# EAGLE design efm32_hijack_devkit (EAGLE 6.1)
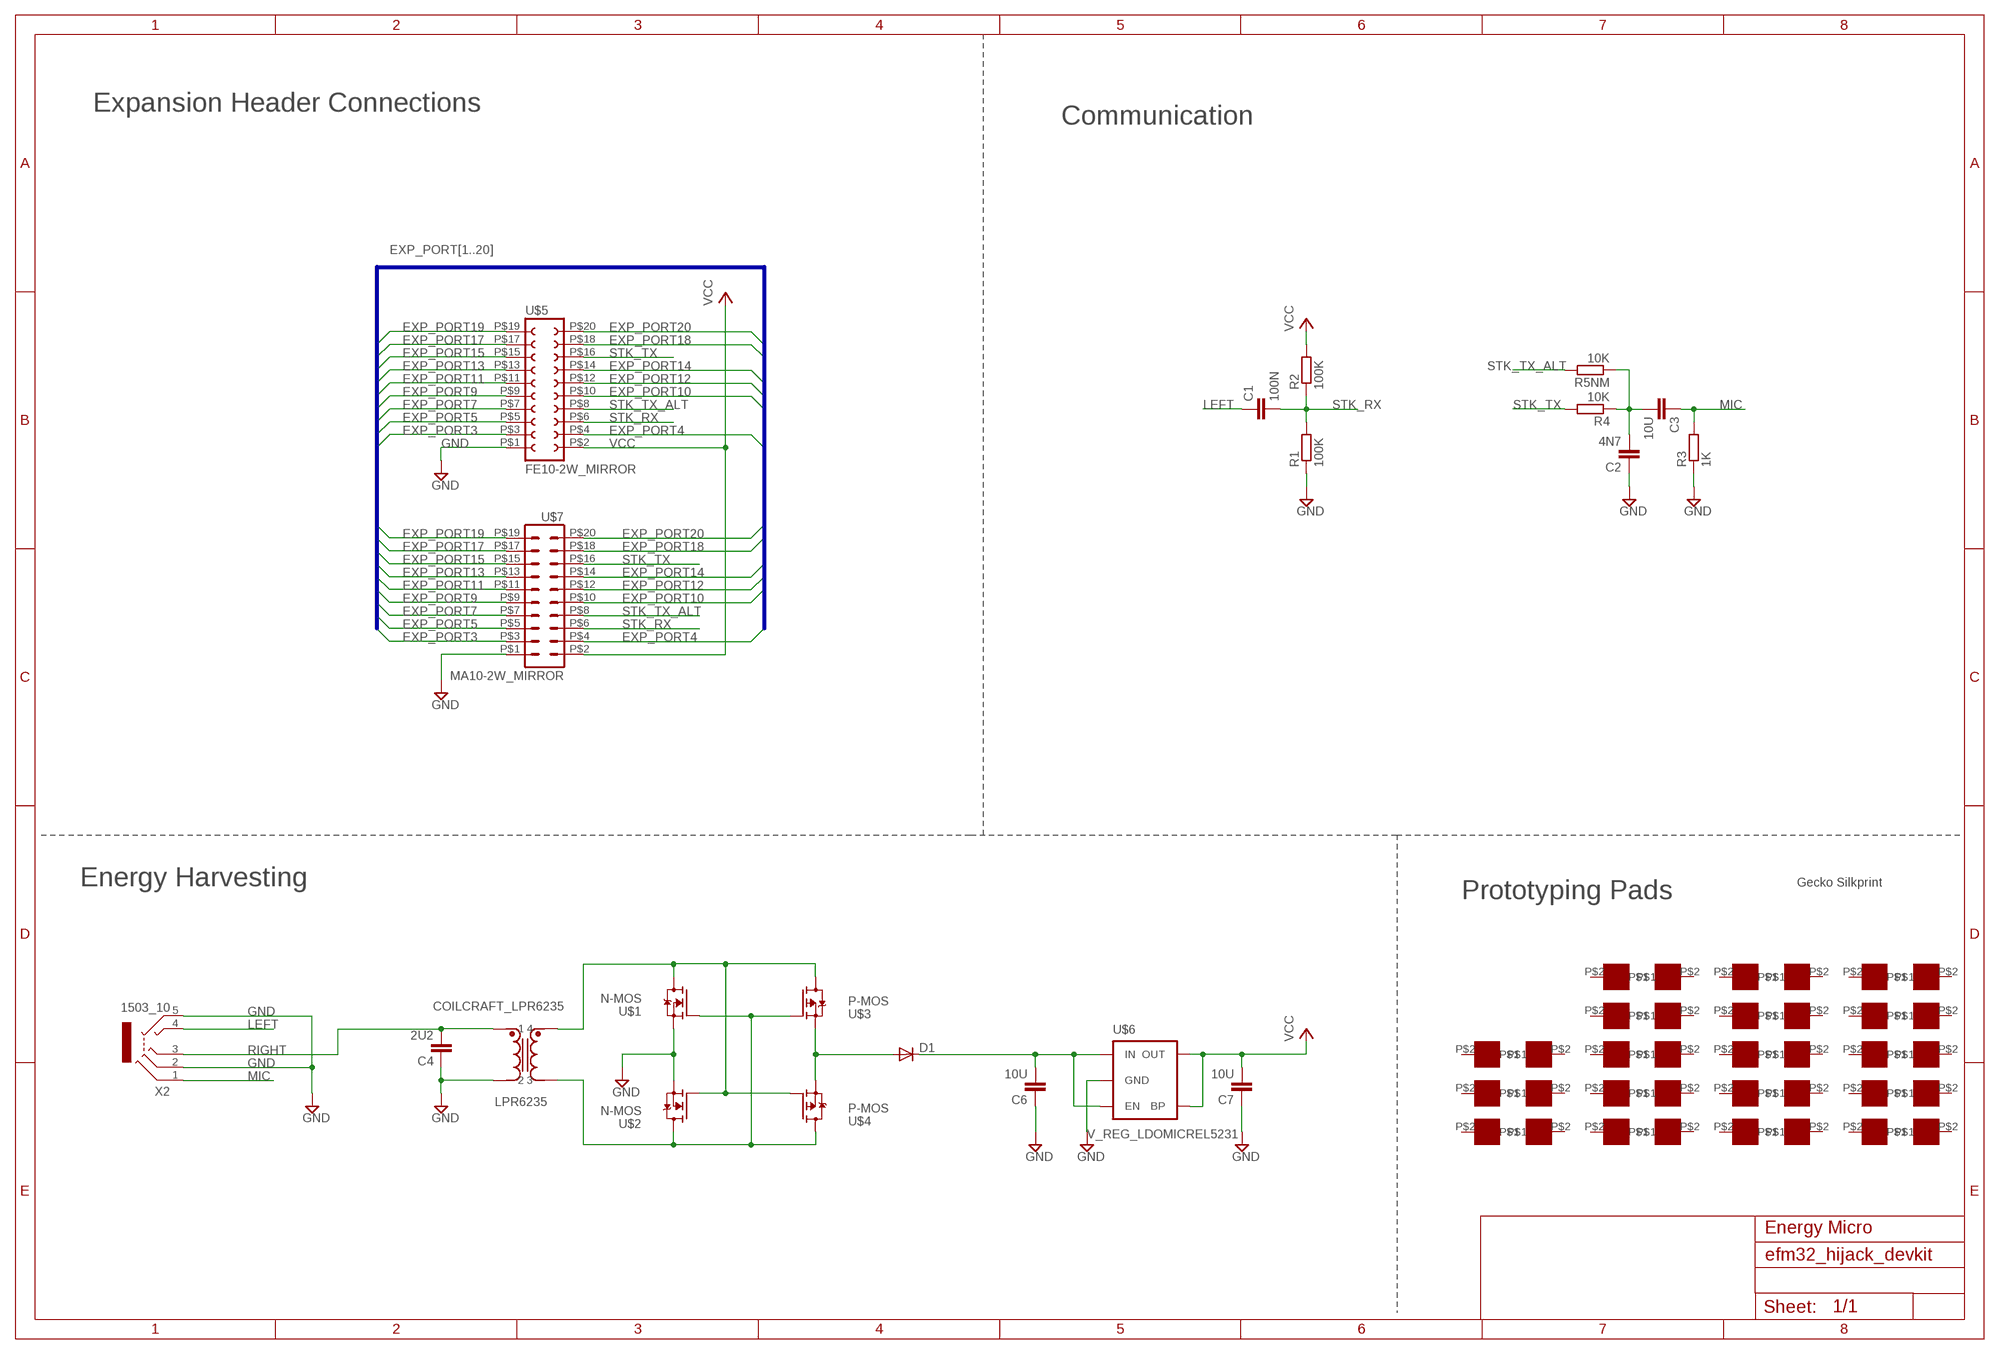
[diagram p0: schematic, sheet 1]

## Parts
C1  100N  C-EUC0603  [C0603]
C2  4N7  C-EUC0603  [C0603]
C3  10U  C-EUC0603  [C0603]
C4  2U2  C-EUC0603  [C0603]
C6  10U  C-EUC0603  [C0603]
C7  10U  C-EUC0603  [C0603]
D1  DIODE-DO214AC  [DO214AC]
LPR6235  COILCRAFT_LPR6235  [COILCRAFT_LPR6235]
R1  100K  R-EU_R0603  [R0603]
R2  100K  R-EU_R0603  [R0603]
R3  1K  R-EU_R0603  [R0603]
R4  10K  R-EU_R0603  [R0603]
R5NM  10K  R-EU_R0603  [R0603]
U$1  N-MOS  [SC-70]
U$2  N-MOS  [SC-70]
U$3  P-MOS  [SC-70]
U$4  P-MOS  [SC-70]
U$5  FE10-2W_MIRROR  [FE10-2W_MIRROR]
U$6  V_REG_LDOMICREL5231  [SOT23-5]
U$7  MA10-2W_MIRROR  [MA10-2W_MIRROR]
U$8  PROTO_PAD  [PROTO_PAD]
U$9  PROTO_PAD  [PROTO_PAD]
U$10  PROTO_PAD  [PROTO_PAD]
U$11  PROTO_PAD  [PROTO_PAD]
U$12  PROTO_PAD  [PROTO_PAD]
U$13  PROTO_PAD  [PROTO_PAD]
U$14  PROTO_PAD  [PROTO_PAD]
U$15  PROTO_PAD  [PROTO_PAD]
U$16  PROTO_PAD  [PROTO_PAD]
U$17  PROTO_PAD  [PROTO_PAD]
U$18  PROTO_PAD  [PROTO_PAD]
U$19  PROTO_PAD  [PROTO_PAD]
U$20  PROTO_PAD  [PROTO_PAD]
U$21  PROTO_PAD  [PROTO_PAD]
U$22  PROTO_PAD  [PROTO_PAD]
U$23  PROTO_PAD  [PROTO_PAD]
U$24  PROTO_PAD  [PROTO_PAD]
U$25  PROTO_PAD  [PROTO_PAD]
U$26  PROTO_PAD  [PROTO_PAD]
U$27  PROTO_PAD  [PROTO_PAD]
U$28  PROTO_PAD  [PROTO_PAD]
U$29  PROTO_PAD  [PROTO_PAD]
U$30  GECKO  [GECKO]
U$32  PROTO_PAD  [PROTO_PAD]
U$33  PROTO_PAD  [PROTO_PAD]
U$36  PROTO_PAD  [PROTO_PAD]
U$37  PROTO_PAD  [PROTO_PAD]
U$38  PROTO_PAD  [PROTO_PAD]
U$39  PROTO_PAD  [PROTO_PAD]
U$40  PROTO_PAD  [PROTO_PAD]
U$41  PROTO_PAD  [PROTO_PAD]
U$42  PROTO_PAD  [PROTO_PAD]
U$43  PROTO_PAD  [PROTO_PAD]
U$44  PROTO_PAD  [PROTO_PAD]
U$45  PROTO_PAD  [PROTO_PAD]
U$46  PROTO_PAD  [PROTO_PAD]
U$47  PROTO_PAD  [PROTO_PAD]
X2  1503_10  [1503_10]

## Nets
EXP_PORT3: U$5.P$3 U$7.P$3
EXP_PORT4: U$5.P$4 U$7.P$4
EXP_PORT5: U$5.P$5 U$7.P$5
EXP_PORT7: U$5.P$7 U$7.P$7
EXP_PORT9: U$5.P$9 U$7.P$9
EXP_PORT10: U$5.P$10 U$7.P$10
EXP_PORT11: U$5.P$11 U$7.P$11
EXP_PORT12: U$5.P$12 U$7.P$12
EXP_PORT13: U$5.P$13 U$7.P$13
EXP_PORT14: U$5.P$14 U$7.P$14
EXP_PORT15: U$5.P$15 U$7.P$15
EXP_PORT17: U$5.P$17 U$7.P$17
EXP_PORT18: U$5.P$18 U$7.P$18
EXP_PORT19: U$5.P$19 U$7.P$19
EXP_PORT20: U$5.P$20 U$7.P$20
GND: C2.1 C4.1 C6.1 C7.1 LPR6235.P$1 R1.1 R3.1 U$1.2(S) U$2.2(S) U$5.P$1 U$6.2(GND) U$7.P$1 X2.2 X2.5
LEFT: C1.1 X2.4
MIC: C3.1 R3.2 X2.1
N$1: C2.2 C3.2 R4.1 R5NM.1
N$13: LPR6235.P$7 U$1.3(D) U$2.1(G) U$3.3(D) U$4.1(G)
N$16: LPR6235.P$4 U$1.1(G) U$2.3(D) U$3.1(G) U$4.3(D)
N$18: D1.A U$3.2(S) U$4.2(S)
N$21: C6.2 D1.C U$6.1(EN) U$6.3(IN)
RIGHT: C4.2 LPR6235.P$10 X2.3
STK_RX: C1.2 R1.2 R2.1 U$5.P$6 U$7.P$6
STK_TX: R4.2 U$5.P$16 U$7.P$16
STK_TX_ALT: R5NM.2 U$5.P$8 U$7.P$8
VCC: C7.2 R2.2 U$5.P$2 U$6.4(OUT) U$6.5(BP) U$7.P$2
Unconnected: U$8.P$2 U$9.P$2 U$10.P$2 U$11.P$2 U$12.P$2 U$13.P$2 U$14.P$2 U$15.P$2 U$16.P$2 U$17.P$2 U$18.P$2 U$19.P$2 U$20.P$2 U$21.P$2 U$22.P$2 U$23.P$2 U$24.P$2 U$25.P$2 U$26.P$2 U$27.P$2 U$28.P$2 U$29.P$2 U$32.P$2 U$33.P$2 U$36.P$2 U$37.P$2 U$38.P$2 U$39.P$2 U$40.P$2 U$41.P$2 U$42.P$2 U$43.P$2 U$44.P$2 U$45.P$2 U$46.P$2 U$47.P$2

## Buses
EXP_PORT[1..20]

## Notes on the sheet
- Expansion Header Connections
- Communication
- Energy Harvesting
- Prototyping Pads
- Energy Micro

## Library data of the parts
C1-C4 C6 C7 = rcl:C-EU: CAPACITOR, European symbol
D1 = diode:DIODE-: DIODE
LPR6235 = trafo:COILCRAFT_LPR6235
R1-R4 R5NM = rcl:R-EU_: RESISTOR, European symbol
U$1 U$2 = transistor-fet:N-MOS
U$3 U$4 = transistor-fet:P-MOS
U$5 = con-lsta:FE10-2W_MIRROR
U$6 = SparkFun_mod:V_REG_LDO: Voltage Regulator LDO Standard 150mA LDO voltage regulator in SOT-23 layout. Micrel part MIC5205. BP (by-pass) pin is used to lower output noise with 470pF cap.
U$7 = con-lstb:MA10-2W_MIRROR
U$8-U$29 U$32 U$33 U$36-U$47 = con-lstb:PROTO_PAD
U$30 = gecko:GECKO
X2 = con-lumberg:1503_10: Jack connectors according to JISC 6560, 3.5 mm Klinkeneinbaukupplung, 3,5 mm, 4-polig/stereo, abgewinkelte Ausführung Source: http://www.lumberg.de/Produkte/PDFs/1503_10.pdf; OC_FARNELL: 1308868; OC_NEWARK: unknown

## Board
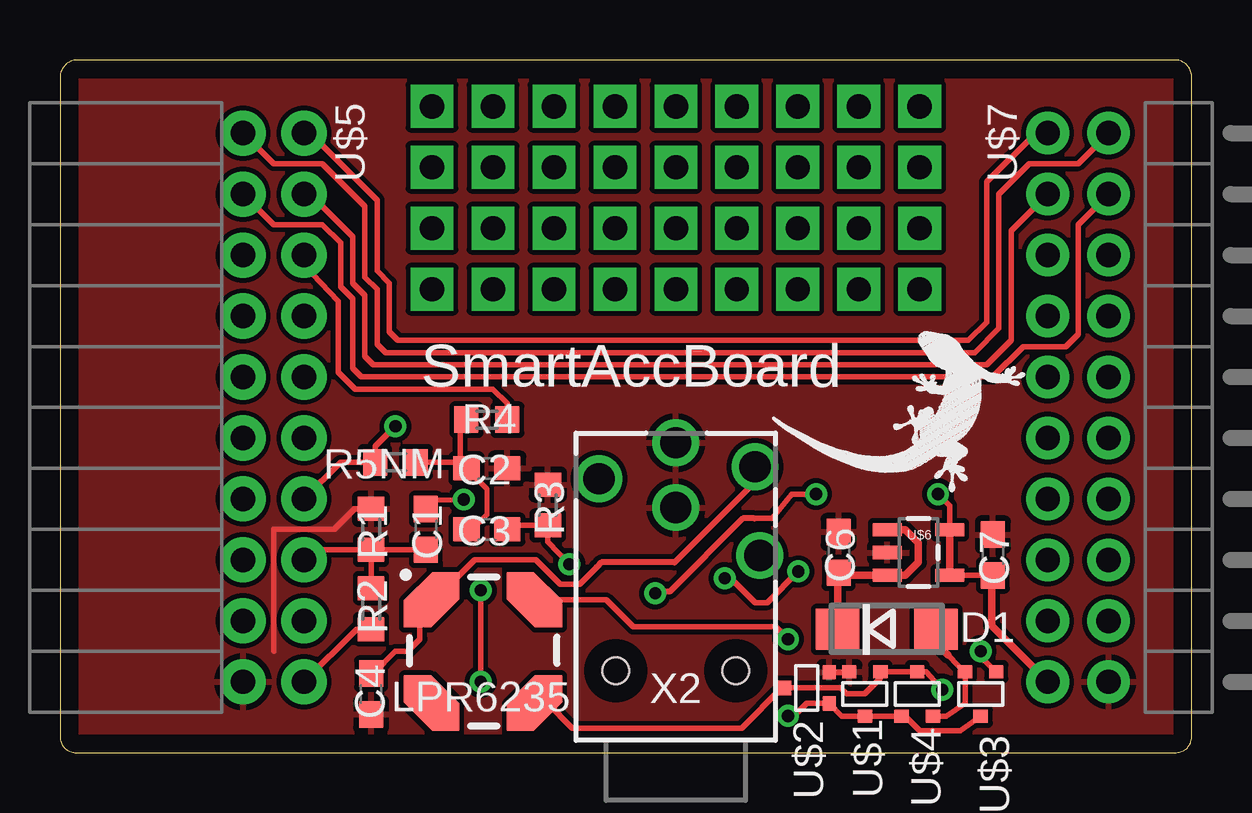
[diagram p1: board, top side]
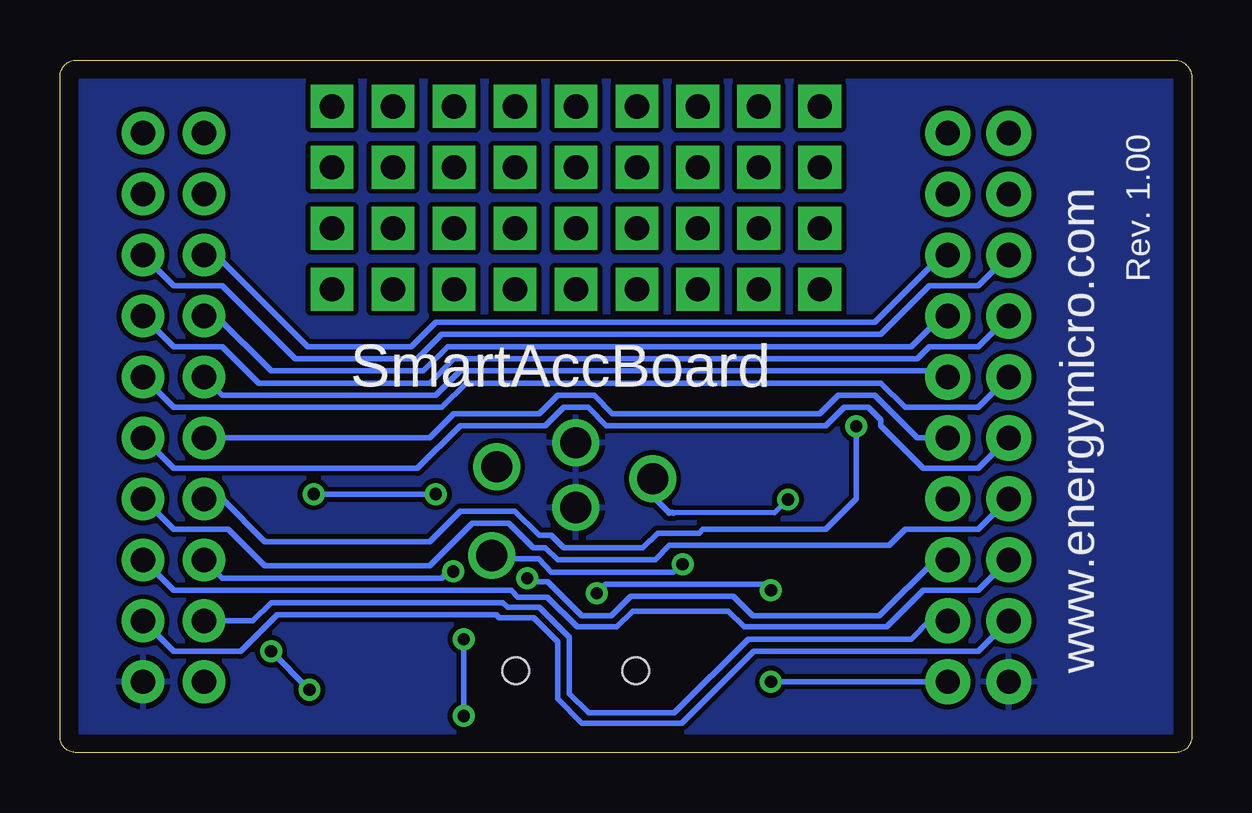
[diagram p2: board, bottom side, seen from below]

Size 47.16 x 28.85 mm. Coordinates in mm from the lower left corner, seen from the top.
Outline: 0.62,0 0.64,0
Outline: 0.64,0 46.51,0 arc90 47.15,0.64 47.15,28.04 arc90 46.54,28.85 0.64,28.85 arc90 0.01,28.02 0.01,0.64 arc90 0.64,0
Copper layers (1*16): Top 0.035mm / dielectric 1.5mm / Bottom 0.035mm
Design rules: minimum track width 8mil, minimum drill 20mil, track to track 8mil, track to pad 8mil, pad to pad 8mil, via to via 8mil, smd to smd 8mil, copper to edge 30mil, drill to drill 8mil, minimum pad ring 10mil, minimum via ring 8mil, stop-mask expansion 4mil, vias tented up to drill 20mil, thermal gap 10mil

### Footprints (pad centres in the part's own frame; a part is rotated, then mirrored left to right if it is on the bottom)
C0603 = smd 1.1 x 1: 1 -0.85,0; 2 0.85,0
DO214AC = smd 1.8 x 1.7: A 2.05,0; C -2.05,0
COILCRAFT_LPR6235 = smd 1.66 x 1.6 rotated 315: P$1 -0.02,1.15 | smd 1.125 x 1.125: P$2 -0.61,1.74; P$3 0.57,0.56; P$5 3.68,0.56; P$6 4.86,1.74; P$8 4.86,4.86; P$9 3.68,6.04; P$11 0.57,6.04; P$12 -0.61,4.86 | smd 1.66 x 1.6 rotated 45: P$4 4.27,1.15 | smd 1.66 x 1.6 rotated 135: P$7 4.27,5.45 | smd 1.66 x 1.6 rotated 225: P$10 -0.02,5.45
R0603 = smd 1 x 1.1: 1 -0.85,0; 2 0.85,0
SC-70 = smd 0.6 x 0.55: 1 -0.65,-0.925; 2 0.65,-0.925; 3 0,0.925
FE10-2W_MIRROR = drill 1.016 pad 1.88: P$1 11.43,-1.27; P$2 11.43,1.27; P$3 8.89,-1.27; P$4 8.89,1.27; P$5 6.35,-1.27; P$6 6.35,1.27; P$7 3.81,-1.27; P$8 3.81,1.27; P$9 1.27,-1.27; P$10 1.27,1.27; P$11 -1.27,-1.27; P$12 -1.27,1.27; P$13 -3.81,-1.27; P$14 -3.81,1.27; P$15 -6.35,-1.27; P$16 -6.35,1.27; P$17 -8.89,-1.27; P$18 -8.89,1.27; P$19 -11.43,-1.27; P$20 -11.43,1.27
SOT23-5 = smd 0.55 x 1.2: 1 -0.95,-1.3; 2 0,-1.3; 3 0.95,-1.3; 4 0.95,1.3; 5 -0.95,1.3
MA10-2W_MIRROR = drill 1.016 pad 1.778: P$1 11.43,1.27; P$2 11.43,-1.27; P$3 8.89,1.27; P$4 8.89,-1.27; P$5 6.35,1.27; P$6 6.35,-1.27; P$7 3.81,1.27; P$8 3.81,-1.27; P$9 1.27,1.27; P$10 1.27,-1.27; P$11 -1.27,1.27; P$12 -1.27,-1.27; P$13 -3.81,1.27; P$14 -3.81,-1.27; P$15 -6.35,1.27; P$16 -6.35,-1.27; P$17 -8.89,1.27; P$18 -8.89,-1.27; P$19 -11.43,1.27; P$20 -11.43,-1.27
PROTO_PAD = drill 1.016 pad 1.778 square: P$2 0,0
1503_10 = drill 1.3 pad 1.9: 1 -3.5,-7.8; 2 0,-9.8; 3 -3.3,-11.5; 4 3.2,-11; 5 0,-12.5 | hole 1.1: -2.5,-3; 2.5,-3

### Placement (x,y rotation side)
C1  15.25,9.3 270 top
C2  17.79,11.84 180 top
C3  17.79,9.3 180 top
C4  12.96,2.44 90 top
C6  32.45,8.34 270 top
C7  38.87,8.23 270 top
D1  34.45,5.13 0 top
LPR6235  15.5,0.91 0 top
R1  12.96,9.3 270 top
R2  12.96,5.99 270 top
R3  20.33,10.31 270 top
R4  17.79,13.87 0 top
R5NM  13.98,12.09 180 top
U$1  33.53,2.44 180 top
U$2  31.12,2.69 90 top
U$3  38.36,2.44 180 top
U$4  35.72,2.44 0 top
U$5  8.9,14.38 270 top
U$6  35.77,8.33 270 top
U$7  42.42,14.38 270 top
U$8  15.5,19.3 0 top
U$9  18.04,19.3 0 top
U$10  15.5,21.84 0 top
U$11  18.04,21.84 0 top
U$12  15.5,24.38 0 top
U$13  18.04,24.38 0 top
U$14  15.5,26.92 0 top
U$15  20.58,19.3 0 top
U$16  23.12,19.3 0 top
U$17  25.66,19.3 0 top
U$18  18.04,26.92 0 top
U$19  23.12,24.38 0 top
U$20  20.58,21.84 0 top
U$21  20.58,24.38 0 top
U$22  23.12,21.84 0 top
U$23  28.2,24.38 0 top
U$24  25.66,24.38 0 top
U$25  25.66,21.84 0 top
U$26  30.74,26.92 0 top
U$27  20.58,26.92 0 top
U$28  30.74,19.3 0 top
U$29  33.28,21.84 0 top
U$30  34.04,14.57 270 top
U$32  28.2,19.3 0 top
U$33  30.74,21.84 0 top
U$36  23.12,26.92 0 top
U$37  25.66,26.92 0 top
U$38  33.28,19.3 0 top
U$39  35.82,19.3 0 top
U$40  28.2,21.84 0 top
U$41  33.28,24.38 0 top
U$42  30.74,24.38 0 top
U$43  35.82,21.84 0 top
U$44  28.2,26.92 0 top
U$45  33.28,26.92 0 top
U$46  35.82,26.92 0 top
U$47  35.82,24.38 0 top
X2  25.66,0.41 180 top

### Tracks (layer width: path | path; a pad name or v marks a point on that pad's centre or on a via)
EXP_PORT3
  Bottom 0.229: U$5.P$3 8.9,4.22 18.24,4.22 21.24,1.22 25.41,1.22 26.42,2.23 26.42,4.62 27.41,5.61 28.86,5.61 28.99,5.74 38.11,5.74 39.63,4.22 42.42,4.22 U$7.P$3
EXP_PORT4
  Bottom 0.229: U$5.P$4 10.93,5.49 11.69,4.72 18.47,4.72 21.57,1.65 25.13,1.65 25.94,2.44 25.94,4.8 27.18,6.04 28.51,6.04 28.71,6.25 38.36,6.25 39.12,5.49 U$7.P$4
EXP_PORT5
  Bottom 0.229: U$5.P$5 8.9,6.76 11.18,6.76 12.71,5.23 18.65,5.23 19.31,5.89 23.3,5.89 23.96,5.23 25.61,5.23 26.85,6.48 28.07,6.48 28.35,6.76 42.42,6.76 U$7.P$5
EXP_PORT7
  Bottom 0.229: U$5.P$7 8.9,9.3 11.94,9.3 12.6,8.64 21.77,8.64 22.36,8.03 26.42,8.03 26.93,8.53 27.44,8.53 28.45,9.55 29.98,9.55 31.76,7.77 38.61,7.77 40.14,9.3 42.42,9.3 U$7.P$7
EXP_PORT9
  Bottom 0.229: U$5.P$9 8.9,11.84 11.18,11.84 12.96,13.61 12.96,13.87 13.47,14.38 14.48,14.38 15.25,13.61 24.39,13.61 25.15,14.38 26.17,14.38 26.93,13.61 30.49,13.61 32.26,11.84 42.42,11.84 U$7.P$9
EXP_PORT10
  Bottom 0.229: U$5.P$10 11.44,13.11 13.21,14.88 14.74,14.88 15.5,14.12 24.14,14.12 24.9,14.88 26.42,14.88 27.18,14.12 30.74,14.12 31.76,13.11 U$7.P$10
EXP_PORT11
  Bottom 0.229: U$5.P$11 8.9,14.38 11.94,14.38 12.96,15.39 30.23,15.39 31.25,14.38 42.42,14.38 U$7.P$11
EXP_PORT12
  Bottom 0.229: U$5.P$12 10.42,15.9 30.49,15.9 31.5,14.88 40.39,14.88 U$7.P$12
EXP_PORT13
  Bottom 0.229: U$5.P$13 8.9,16.92 10.93,16.92 11.44,16.41 30.74,16.41 31.76,15.39 38.87,15.39 40.39,16.92 42.42,16.92 U$7.P$13
EXP_PORT14
  Bottom 0.229: U$5.P$14 10.42,18.19 11.69,16.92 30.99,16.92 32.01,15.9 38.36,15.9 40.65,18.19 U$7.P$14
EXP_PORT15
  Bottom 0.229: U$5.P$15 8.9,19.46 10.93,19.46 12.96,17.42 31.25,17.42 32.26,16.41 37.34,16.41 40.39,19.46 42.42,19.46 U$7.P$15
EXP_PORT17
  Top 0.229: U$5.P$17 8.9,22 10.93,22 11.69,21.23 11.69,19.41 12.2,18.9 12.2,16 12.55,15.65 38.87,15.65 40.14,16.92 41.92,16.92 42.42,17.42 42.42,22 U$7.P$17
EXP_PORT18
  Top 0.229: U$5.P$18 10.42,23.27 12.2,21.49 12.2,19.56 12.71,19.05 12.71,16.51 13.06,16.15 38.61,16.15 39.63,17.17 39.63,21.74 U$7.P$18
EXP_PORT19
  Top 0.229: U$5.P$19 8.9,24.54 10.93,24.54 12.71,22.76 12.71,19.81 13.21,19.3 13.21,17.02 13.57,16.66 38.11,16.66 39.12,17.68 39.12,23.27 40.39,24.54 42.42,24.54 U$7.P$19
EXP_PORT20
  Top 0.229: U$5.P$20 10.42,25.81 13.21,23.01 13.21,20.07 13.72,19.56 13.72,17.53 14.08,17.17 37.85,17.17 38.61,17.93 38.61,23.77 40.65,25.81 U$7.P$20
GND
  Top 0.229: U$2.2 32.86,3.34 U$1.2 | R1.1 12.29,10.15 11.44,9.3 8.9,9.3 8.9,4.22
  pour Bottom: 47.25,28.75 47.25,0 0.01,0 0.01,28.85
  pour Top: 0.01,28.75 47.25,28.75 47.25,0 0.01,0
LEFT  (via drill 0.51)
  Top 0.203: C1.1 15.64,10.54 v16.82,10.54
  Bottom 0.203: 21.6,9.98 17.38,9.98 v16.82,10.54
  Bottom 0.254: 21.6,9.98 21.77,9.98 22.36,10.57 22.36,11.3 X2.4
MIC  (via drill 0.51)
  Top 0.229: C3.1 18.8,9.46 R3.2 20.33,8.79 v21.22,7.85
  Bottom 0.229: v21.22,7.85 21.6,7.52 26.68,7.52 27.21,8.08 29.01,8.08 X2.1
N$1
  Top 0.203: C3.2 17.18,9.3 17.79,9.91 17.79,10.99 C2.2
  Top 0.229: R5NM.1 16.68,12.09 | 16.68,12.09 C2.2 | 16.68,12.09 16.68,13.61 R4.1
N$13  (via drill 0.51)
  Top 0.229: U$3.3 37.51,0.91 35.82,0.91 35.22,1.51 U$4.1 U$1.3 32.58,1.51 U$2.1 31.11,2.04 30.74,1.68 30.49,1.68 v30.33,1.52 | LPR6235.P$7 22.75,6.36 23.88,5.23 29.83,5.23 v30.33,4.72
  Bottom 0.229: v30.33,4.72 v30.33,1.52
N$16  (via drill 0.51)
  Top 0.229: v36.76,2.62 36.09,3.36 U$4.3 U$1.1 34.18,3.09 33.53,2.44 32.77,2.44 32.52,2.69 U$2.3 30.08,2.69 28.4,1.02 21.34,1.02 20.29,2.06 LPR6235.P$4 | v38.36,4.22 38.36,3.96 U$3.1
  Bottom 0.229: v36.76,2.62 v38.36,4.22
N$18
  Top 0.229: U$4.2 36.93,1.51 37.71,2.04 U$3.2 37.46,3.6 36.99,4.06 36.84,4.22
  Top 0.305: D1.A 36.5,4.55 36.58,4.47 36.79,4.27 36.99,4.06
N$21
  Top 0.305: D1.C 32.4,7.44 C6.2 32.55,7.38 U$6.3 35.23,7.38 35.77,7.92 35.77,8.74 35.23,9.28 U$6.1
RIGHT
  Top 0.229: C4.2 13.05,3.29 13.98,4.22 14.48,4.22 14.99,4.72 14.99,5.88 LPR6235.P$10 15.62,6.36 17.28,8.03 19.82,8.03 20.83,7.01 21.65,7.01 22.36,7.72 22.46,7.82
  Top 0.254: X2.3 28.96,11.28 25.61,7.92 22.56,7.92 22.36,7.72
STK_RX  (via drill 0.51)
  Top 0.229: R1.2 R2.1 | R1.2 10.59,8.45 U$5.P$6 | R1.2 C1.2 | v27.69,7.26 27.95,7.26 28.96,6.25 29.47,6.25 v30.77,7.54
  Bottom 0.229: U$5.P$6 10.67,8.03 13.01,5.69 18.29,5.69 19.11,6.5 23.37,6.5 24.19,5.69 25.41,5.69 26.83,7.11 27.54,7.11 v27.69,7.26 | v30.77,7.54 30.99,7.52 31.25,7.26 40.39,7.26 U$7.P$6
STK_TX
  Top 0.229: R4.2 18.64,14.54 18.04,15.14 12.3,15.14 11.59,15.85 11.59,18.8 10.17,20.32 U$5.P$16
  Bottom 0.229: U$5.P$16 10.42,20.73 13.21,17.93 31.5,17.93 32.52,16.92 36.84,16.92 40.65,20.73 U$7.P$16
STK_TX_ALT  (via drill 0.51)
  Top 0.229: U$5.P$8 11.69,12.09 R5NM.2 13.13,12.76 v13.98,13.59
  Bottom 0.229: v13.98,13.59 13.98,10.57 15.25,9.3 20.38,9.3 20.53,9.14 22.26,9.14 22.87,8.53 26.17,8.53 26.68,9.04 27.18,9.04 28.2,10.06 30.49,10.06 31.76,8.79 38.61,8.79 40.39,10.57 U$7.P$8
VCC  (via drill 0.51)
  Top 0.229: R2.2 12.36,5.14 U$5.P$2 | v17.53,2.95 v17.53,6.76 | 37.19,7.32 37,7.32 | C7.2 U$6.4 37,7.32 | U$6.5 37.07,10.28 v36.58,10.77 | v31.5,10.77 30.49,10.77 29.67,9.75 28.94,9.75 | 36.99,7.32 37,7.32
  Top 0.254: 28.94,9.75 28.45,9.75 25.41,6.71 24.87,6.71 v24.8,6.63
  Top 0.305: U$7.P$2 38.82,5.28 38.82,7.33 C7.2 | U$6.4 U$6.5
  Bottom 0.229: v17.53,6.76 17.79,7.01 24.42,7.01 v24.8,6.63 | U$5.P$2 v17.53,2.95 | v36.58,10.77 v31.5,10.77

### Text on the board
tValues: NM
_tsilk: SmartAccBoard
_bsilk: Rev. 1.00 | SmartAccBoard | www.energymicro.com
